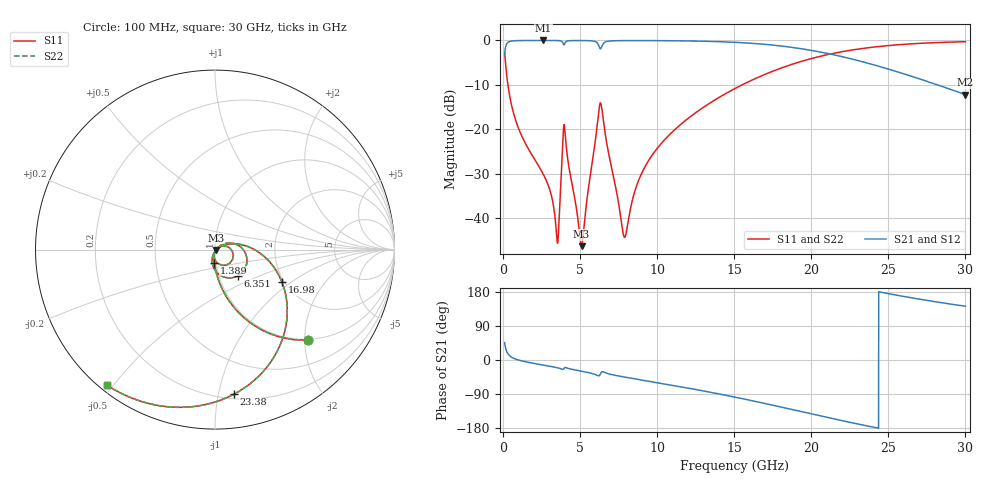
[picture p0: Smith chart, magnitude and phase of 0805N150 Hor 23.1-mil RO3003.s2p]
# GHz S MA R 50
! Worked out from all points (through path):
!   3201 points, 100 MHz to 30 GHz, reference 50 ohm
!   highest |S21| = -0.02 dB at 2.604 GHz (marker M1); lowest = -12.2 dB at 30 GHz (marker M2)
!   group delay of S21, straight-line fit = 21.7 ps
!   lowest |S11| = -46.3 dB at 5.09 GHz (marker M3), VSWR 1.01, Z = 50.4 - j0.27 ohm
!   |S11| at or under -10 dB: 315 MHz to 15.52 GHz (15.2 GHz wide, 192 % of centre)
!   |S22| runs from -46.3 to -0.3 dB; largest |S21 - S12| = 0
!   S11 on the Smith chart (normalised r, x): 100 MHz: 0.98, -2.08; 1.389 GHz: 0.98, -0.14; 6.351 GHz: 1.23, -0.37; 16.98 GHz: 1.95, -0.84; 23.38 GHz: 0.23, -1.11; 30 GHz: 0.02, -0.48
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0.1  0.7245 -44.1  0.6888 45.8  0.6888 45.8  0.7245 -44.1
0.4270312  0.2384 -78.6  0.9705 11.3  0.9705 11.3  0.2384 -78.6
1.389438  0.07263 -93.0  0.996 -4.0  0.996 -4.0  0.07263 -93.0
2.604125  0.03136 -100.0  0.9975 -13.5  0.9975 -13.5  0.03136 -100.0
3.108687  0.01872 -99.5  0.9972 -17.1  0.9972 -17.1  0.01872 -99.5
3.510469  0.005472 -51.7  0.9952 -20.3  0.9952 -20.3  0.005472 -51.7
3.641281  0.01039 20.8  0.9922 -21.7  0.9922 -21.7  0.01039 20.8
3.874875  0.07336 11.7  0.9402 -25.1  0.9402 -25.1  0.07336 11.7
4.015031  0.09494 -65.9  0.9321 -19.5  0.9321 -19.5  0.09494 -65.9
5.089563  0.004839 -33.6  0.995 -29.5  0.995 -29.5  0.004839 -33.6
6.042625  0.08892 24.5  0.9575 -39.5  0.9575 -39.5  0.08892 24.5
6.350969  0.1941 -48.5  0.8109 -33.8  0.8109 -33.8  0.1941 -48.5
6.678  0.07831 -100.9  0.966 -34.3  0.966 -34.3  0.07831 -100.9
7.874  0.006081 -44.3  0.9936 -45.0  0.9936 -45.0  0.006081 -44.3
8.789687  0.02644 27.4  0.9942 -51.4  0.9942 -51.4  0.02644 27.4
10.06978  0.06303 25.2  0.9926 -60.2  0.9926 -60.2  0.06303 25.2
15.05  0.2875 -9.4  0.9504 -98.0  0.9504 -98.0  0.2875 -9.4
16.98416  0.4136 -25.8  0.902 -114.7  0.902 -114.7  0.4136 -25.8
20.03956  0.6265 -53.3  0.7695 -142.5  0.7695 -142.5  0.6265 -53.3
23.37528  0.8128 -82.6  0.5715 -171.9  0.5715 -171.9  0.8128 -82.6
25.01978  0.8741 -95.7  0.4743 175.0  0.4743 175.0  0.8741 -95.7
30  0.9659 -128.7  0.2455 141.9  0.2455 141.9  0.9659 -128.7
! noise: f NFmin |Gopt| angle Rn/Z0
0.1  0.0006181  0.9008  0.9181  0.001363
3.417  0.008502  0.7719  19.97  0.007377
6.743  0.03043  0.8705  38.81  0.04506
10.06  0.01667  0.692  56.34  0.008273
13.39  0.021  0.688  72.53  0.008662
16.7  0.02674  0.7036  87.4  0.009507
20.03  0.03421  0.7296  101.2  0.01051
23.35  0.0443  0.763  114.3  0.01166
26.67  0.05875  0.8024  126.9  0.01294
30  0.08071  0.845  139.3  0.01409
